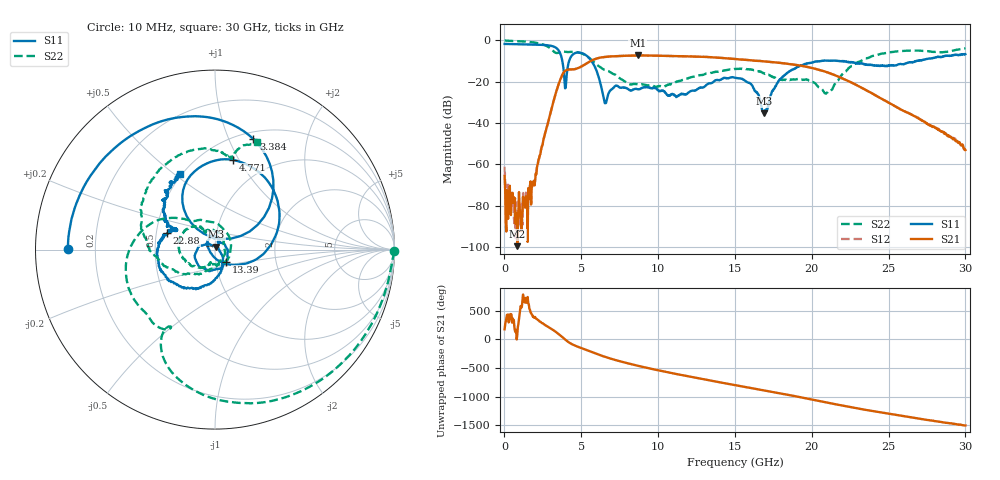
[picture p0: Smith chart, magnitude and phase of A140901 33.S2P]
!  2-Port S-parameters saved by WinCal
! VAR MeasName=S-Parameters (CALIBRATED_DATA) read from VNA (N5244A)
! VAR MeasDate=11/3/2014 9:29:32 AM
! VAR NAME=A140901 33
! VAR FILENAME=A140901 33.S2P
! VAR DATE=11/3/2014 9:29:32 AM
! VAR PHYS_PORTS=1,2
# Hz S RI R 50
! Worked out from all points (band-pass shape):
!   801 points, 10 MHz to 30 GHz, reference 50 ohm
!   highest |S21| = -7.24 dB at 8.67 GHz (marker M1); lowest = -99.5 dB at 834.7 MHz (marker M2)
!   |S21| within 3 dB of the highest: 5.549 GHz to 17.02 GHz (11.48 GHz wide, 102 % of centre); 17.05969 GHz to 17.06865 GHz (8.957 MHz wide, 0.0525 % of centre)
!   lowest |S11| = -35.2 dB at 16.88 GHz (marker M3), VSWR 1.04, Z = 50.7 + j1.6 ohm
!   |S11| at or under -10 dB: 3.767 GHz to 4.206 GHz (439.2 MHz wide, 11 % of centre); 5.667 GHz to 20.55 GHz (14.89 GHz wide, 114 % of centre); 22.1 GHz to 26.76 GHz (4.668 GHz wide, 19.1 % of centre)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
!   |S22| runs from -25.8 to 0.0 dB; largest |S21 - S12| = 0.0033
!   S11 on the Smith chart (normalised r, x): 10 MHz: 0.10, +0.00; 3.384 GHz: 0.58, +1.24; 4.771 GHz: 0.70, +0.95; 13.39 GHz: 1.12, -0.15; 22.88 GHz: 0.57, +0.11; 30 GHz: 0.49, +0.53
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1e7  -0.8205 0.00269  -0.000527 3.23e-05  -0.000335 -0.000818  0.9972 -0.00926
2.724125e8  -0.8137 0.0892  6.96e-05 -0.000134  5.71e-05 0.000121  0.9646 -0.1773
8.34725e8  -0.7682 0.2677  2.36e-06 1.03e-05  2.28e-05 -0.000122  0.8249 -0.4916
1.884375e9  -0.5599 0.565  0.000292 0.000252  0.000223 0.000299  0.2921 -0.8478
3.383875e9  0.2144 0.6153  -0.0327 0.0501  -0.0328 0.0499  -0.2508 -0.4279
3.983675e9  -0.016 0.0694  0.1837 -0.0376  0.1836 -0.0372  -0.362 -0.3865
4.770912e9  0.1027 0.4992  -0.1314 -0.1673  -0.131 -0.1669  -0.4958 -0.1396
5.033325e9  0.259 0.419  -0.2146 -0.0995  -0.2141 -0.1004  -0.483 -0.0187
6.570312e9  -0.0264 -0.0152  0.2425 0.3162  0.2425 0.3161  -0.1035 0.1613
7.470012e9  -0.00917 0.0739  0.3969 -0.139  0.3973 -0.1387  0.045 0.1156
8.669612e9  -0.011 0.0653  -0.0829 -0.4266  -0.0827 -0.4262  0.0574 -0.0662
1.001916e10  0.0167 0.0592  -0.4275 0.0117  -0.4263 0.0115  -0.0256 -0.0737
1.163112e10  0.026 0.0441  -0.00944 0.4138  -0.0101 0.4136  -0.0562 -0.0962
1.339304e10  0.0631 -0.0665  0.3931 0.00432  0.3933 0.00535  -0.1402 -0.0808
1.5005e10  -0.0979 -0.0777  0.0652 -0.349  0.065 -0.3491  -0.2014 0.0179
1.687938e10  0.00715 0.0158  -0.3071 -0.05  -0.3081 -0.0511  -0.098 0.1285
1.796651e10  0.0378 -0.1091  -0.2012 0.2009  -0.203 0.2018  -0.0539 0.0973
2.002832e10  -0.224 -0.1872  0.1907 0.0978  0.1915 0.098  0.0152 0.0974
2.1003e10  -0.3114 -0.0864  0.1538 -0.0724  0.1523 -0.0735  0.055 -0.00332
2.287738e10  -0.2657 0.0917  -0.0451 -0.0716  -0.0444 -0.0713  -0.2631 -0.0994
2.501416e10  -0.2139 0.1128  -0.0238 0.02  -0.0237 0.0202  -0.3753 0.3487
3e10  -0.194 0.4214  0.000934 -0.00202  0.000782 -0.00212  0.2338 0.5987
